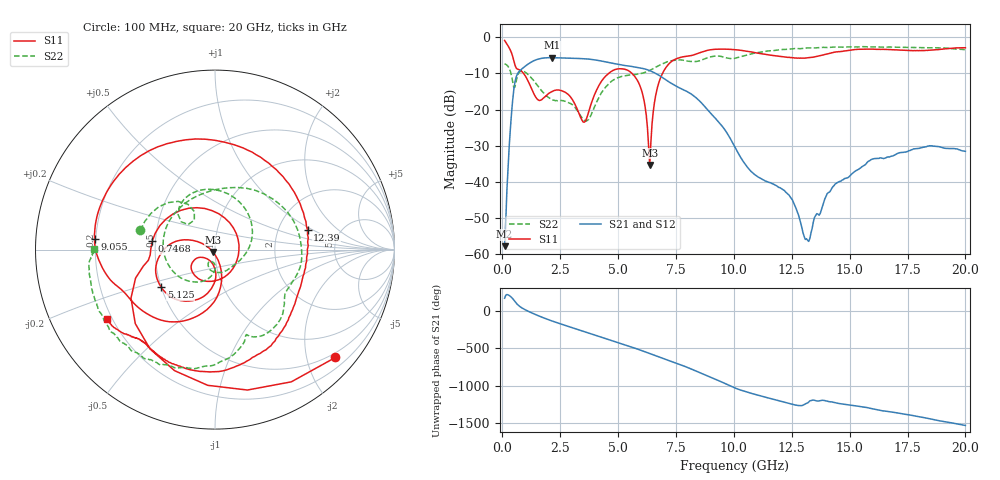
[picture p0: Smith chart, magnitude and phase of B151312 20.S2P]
!  2-Port S-parameters saved by WinCal
! VAR MeasName=S-Parameters (CALIBRATED_DATA) read from VNA (N5244A)
! VAR MeasDate=12/8/2015 5:45:00 PM
! VAR NAME=B151312 20
! VAR FILENAME=B151312 20.S2P
! VAR DATE=12/8/2015 5:45:00 PM
! VAR PHYS_PORTS=1,2
# Hz S DB R 50
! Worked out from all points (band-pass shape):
!   401 points, 100 MHz to 20 GHz, reference 50 ohm
!   highest |S21| = -5.67 dB at 2.14 GHz (marker M1); lowest = -57.8 dB at 100 MHz (marker M2)
!   |S21| within 3 dB of the highest: 865.2 MHz to 6.076 GHz (5.211 GHz wide, 150 % of centre)
!   lowest |S11| = -35.3 dB at 6.369 GHz (marker M3), VSWR 1.03, Z = 48.9 - j1.26 ohm
!   |S11| at or under -10 dB: 914.6 MHz to 4.598 GHz (3.683 GHz wide, 134 % of centre); 5.597 GHz to 6.919 GHz (1.322 GHz wide, 21.1 % of centre)
!   |S22| runs from -23.2 to -2.6 dB; largest |S21 - S12| = 0.0016
!   S11 on the Smith chart (normalised r, x): 100 MHz: 0.40, -2.56; 746.8 MHz: 0.48, +0.05; 5.125 GHz: 0.50, -0.24; 9.055 GHz: 0.20, +0.04; 12.39 GHz: 2.93, +0.89; 20 GHz: 0.18, -0.29
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1e8  -0.91 -41.9  -57.77 163.9  -57.85 162.7  -7.36 165.6
4.4825e8  -5.34 -150.0  -17.42 158.7  -17.42 158.7  -12.36 118.5
7.4675e8  -9.05 172.3  -9.35 56.2  -9.35 56.2  -9.60 121.0
1.294e9  -14.69 72.9  -6.73 -34.1  -6.73 -34.1  -11.53 43.7
2.13975e9  -15.04 -95.1  -5.67 -137.7  -5.66 -137.7  -17.19 -37.4
2.73675e9  -15.30 -140.0  -5.79 160.3  -5.79 160.3  -17.76 -81.5
3.43325e9  -22.84 -139.2  -5.93 90.7  -5.93 90.7  -22.20 -116.7
4.22925e9  -12.74 -97.4  -6.53 10.2  -6.53 10.2  -15.99 -100.9
5.12475e9  -8.74 -144.9  -7.65 -78.7  -7.63 -78.7  -10.90 -176.2
5.92075e9  -13.06 168.0  -8.47 -161.3  -8.46 -161.4  -10.13 114.4
6.3685e9  -35.30 -131.3  -9.25 147.7  -9.25 147.7  -9.20 80.8
6.7665e9  -12.43 -84.6  -10.53 101.4  -10.53 101.4  -7.83 52.1
7.61225e9  -5.75 -134.8  -13.89 8.0  -13.85 7.9  -6.28 -5.0
9.055e9  -3.43 175.1  -21.43 -174.4  -21.44 -175.0  -5.34 -50.2
1.005e10  -3.46 132.9  -30.41 49.3  -30.45 49.0  -5.82 -70.6
1.11445e10  -4.53 79.6  -39.00 -55.0  -39.06 -54.8  -4.17 -85.6
1.238825e10  -5.56 12.0  -43.68 -156.6  -43.78 -156.3  -3.34 -105.3
1.31345e10  -5.75 -20.5  -55.71 -155.1  -55.59 -154.3  -2.99 -115.2
1.338325e10  -5.58 -29.6  -52.82 -112.9  -52.68 -114.2  -2.99 -117.7
1.437825e10  -4.13 -61.3  -40.57 -145.7  -40.56 -145.6  -2.72 -129.6
1.67165e10  -3.44 -114.6  -33.12 93.7  -32.95 93.7  -2.72 -152.4
2e10  -2.93 -147.2  -31.56 -89.1  -31.63 -90.4  -3.45 179.8
